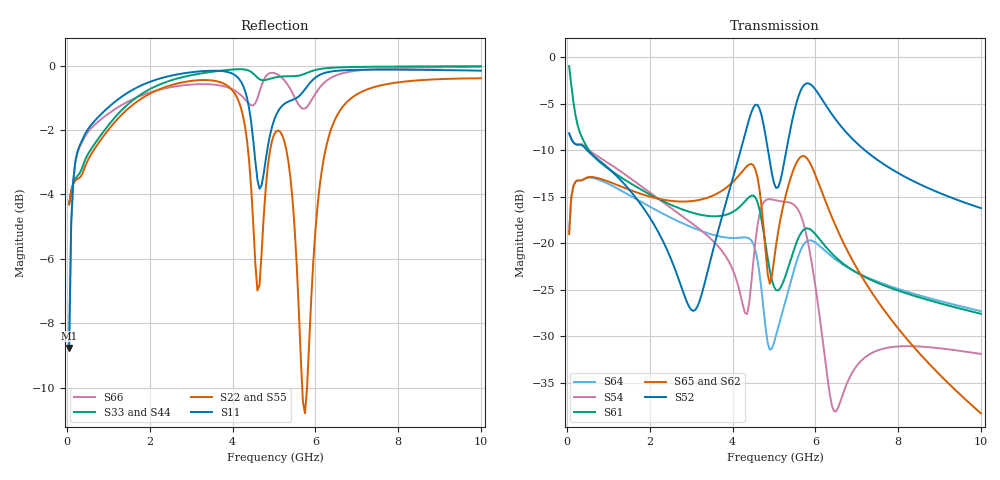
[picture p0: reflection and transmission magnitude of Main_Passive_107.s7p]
! Created Tue Jun  9 07:00:21 2020
# ghz S ma R 50
! 7 Port Network Data from SP1.SP block
! freq  magS11  angS11  magS12  angS12  magS13  angS13  magS14  angS14
!  magS15  angS15  magS16  angS16  magS17  angS17
!  magS21  angS21
!  magS22  angS22  magS23  angS23  magS24  angS24  magS25  angS25
!  magS26  angS26  magS27  angS27
!  magS31  angS31  magS32  angS32
!  magS33  angS33  magS34  angS34  magS35  angS35  magS36  angS36
!  magS37  angS37
!  magS41  angS41  magS42  angS42  magS43  angS43
!  magS44  angS44  magS45  angS45  magS46  angS46  magS47  angS47
!  magS51  angS51  magS52  angS52  magS53  angS53  magS54  angS54
!  magS55  angS55  magS56  angS56  magS57  angS57
!  magS61  angS61
!  magS62  angS62  magS63  angS63  magS64  angS64  magS65  angS65
!  magS66  angS66  magS67  angS67
!  magS71  angS71  magS72  angS72
!  magS73  angS73  magS74  angS74  magS75  angS75  magS76  angS76
!  magS77  angS77
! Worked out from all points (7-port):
!   200 points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, 50 MHz to 10 GHz, reference 50 ohm
!   strongest paths, dB at 50 MHz, 2.55 GHz, 5.05 GHz, 7.55 GHz, 10 GHz:
!     S52: -8.2, -22.1, -14.1, -11.2, -16.2
!     S65: -19.0, -15.5, -20.2, -26.5, -38.3
!     S62: -19.0, -15.5, -20.5, -26.6, -38.4
!     S61: -1.0, -15.9, -25.0, -24.3, -27.6
!     S54: -8.2, -16.3, -15.4, -31.4, -31.9
!     S64: -19.0, -17.3, -29.9, -24.2, -27.3
!   lowest |S11| = -8.8 dB at 50 MHz (marker M1), VSWR 2.15, Z = 29.5 - j22.1 ohm
!   |S11| at or under -10 dB: nowhere
